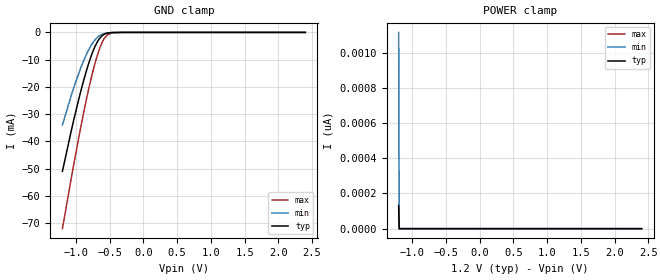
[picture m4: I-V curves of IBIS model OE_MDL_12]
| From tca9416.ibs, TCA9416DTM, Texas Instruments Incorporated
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[Model]   OE_MDL_12
Model_type   Input
Vinl = 0.420
Vinh = 0.780
|   typ   min   max
C_comp   2pF   1.95pF   2.13pF
[Voltage Range]   1.2   1.08   1.32
[Temperature Range]   27   125   -40
[Power Clamp Reference]   1.2   1.08   1.32
[GND Clamp Reference]   0   0   0
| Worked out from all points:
|   GND clamp passes 1 mA (typ) near -0.60 V on its own axis
[GND Clamp]
|OE_MDL_12
|   Voltage   I(typ)   I(min)   I(max)
-1.2V     -51mA      -33.94mA   -72.04mA
-1.027V   -31.63mA   -19.97mA   -47.83mA
-922.8mV  -21.12mA   -12.71mA   -34.1mA
-818.4mV  -11.99mA   -6.75mA    -21.59mA
-750mV    -7.092mA   -3.819mA   -14.43mA
-674.4mV  -3.136mA   -1.666mA   -7.775mA
-609.6mV  -1.174mA   -674.7uA   -3.555mA
-580.8mV  -687.5uA   -425.8uA   -2.247mA
-537.6mV  -277uA     -199.6uA   -965.1uA
-465.6mV  -48.41uA   -47.04uA   -159.7uA
-300mV    -351.3nA   -908.3nA   -499.1nA
2.4V      0A         0A         0A
[POWER Clamp]
|OE_MDL_12
|   Voltage   I(typ)   I(min)   I(max)
-1.2V     131.1pA    1.116nA    70.18pA
-1.193V   0A         0A         0A
-1.189V   0A         0A         0A
2.4V      0A         0A         0A
